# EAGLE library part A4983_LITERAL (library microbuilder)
A4983 2A Micro-Stepping Stepper Motor Driver Logic: 3.0-5.5V Load Supply: 8.0-35V
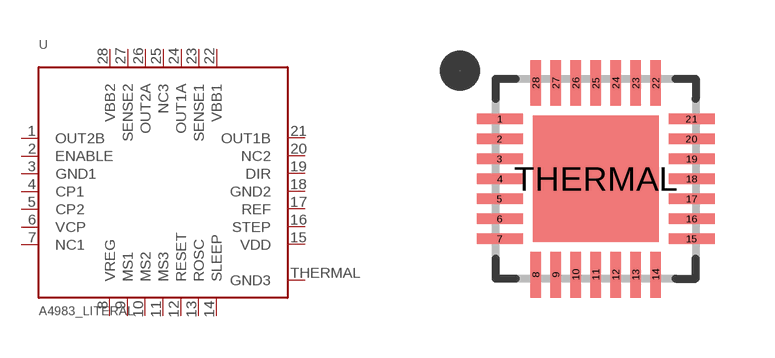
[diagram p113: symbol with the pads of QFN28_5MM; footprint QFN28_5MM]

Designator prefix U

## A4983_LITERAL  [QFN28_5MM]
1  OUT2B
2  ENABLE  in
3  GND1  pwr
4  CP1
5  CP2
6  VCP
7  NC1  nc
8  VREG
9  MS1  in
10  MS2  in
11  MS3  in
12  RESET  in
13  ROSC
14  SLEEP
15  VDD  pwr
16  STEP  in
17  REF
18  GND2  pwr
19  DIR  in
20  NC2  nc
21  OUT1B
22  VBB1
23  SENSE1
24  OUT1A
25  NC3  nc
26  OUT2A
27  SENSE2
28  VBB2
THERMAL  GND3  pwr

## Footprint QFN28_5MM (pad centres in mm)
28-Pin 0.5mm pitch QFN (5.0x5.0mm) Source: http://www.allegromicro.com/en/Products/Part_Numbers/4983/4983.pdf
smd 1.15 x 0.27: 1 -2.4,1.5; 2 -2.4,1; 3 -2.4,0.5; 4 -2.4,0; 5 -2.4,-0.5; 6 -2.4,-1; 7 -2.4,-1.5; 15 2.4,-1.5; 16 2.4,-1; 17 2.4,-0.5; 18 2.4,0; 19 2.4,0.5; 20 2.4,1; 21 2.4,1.5
smd 0.27 x 1.15: 8 -1.5,-2.4; 9 -1,-2.4; 10 -0.5,-2.4; 11 0,-2.4; 12 0.5,-2.4; 13 1,-2.4; 14 1.5,-2.4; 22 1.5,2.4; 23 1,2.4; 24 0.5,2.4; 25 0,2.4; 26 -0.5,2.4; 27 -1,2.4; 28 -1.5,2.4
smd 3.15 x 3.15: THERMAL 0,0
